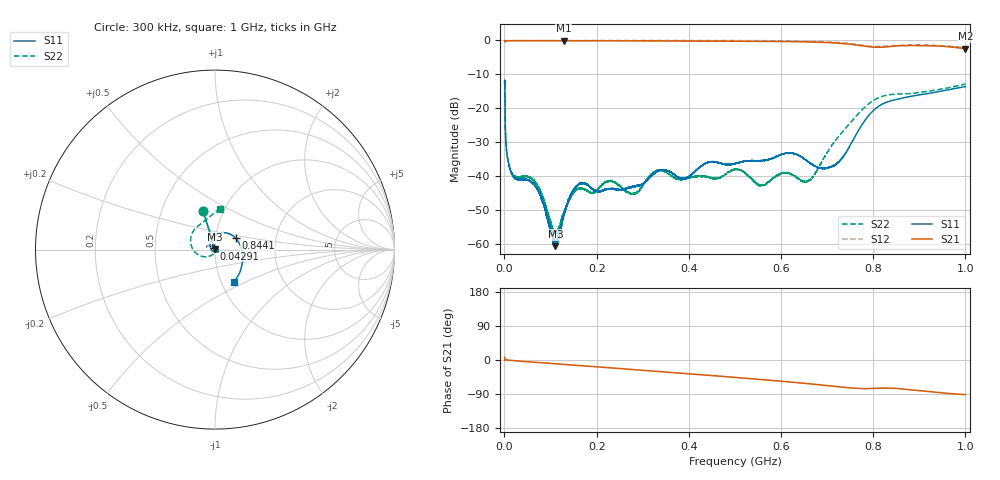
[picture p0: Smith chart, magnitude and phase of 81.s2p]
!Keysight Technologies,N5232A,MY52221221,A.10.65.11
!Date: Thursday, June 15, 2023 18:07:57
!Correction: S11(Full 2 Port(1,4))
!S41(Full 2 Port(1,4))
!S14(Full 2 Port(1,4))
!S44(Full 2 Port(1,4))
!S2P File: Measurements: S11, S41, S14, S44:
# Hz S  RI  R 50
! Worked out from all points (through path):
!   16001 points, 300 kHz to 1 GHz, reference 50 ohm
!   highest |S21| = -0.10 dB at 128.2 MHz (marker M1); lowest = -2.5 dB at 999.9 MHz (marker M2)
!   group delay of S21, straight-line fit = 257 ps
!   lowest |S11| = -60.7 dB at 110.5 MHz (marker M3), VSWR 1.00, Z = 50 + j0.0882 ohm
!   |S11| at or under -10 dB: start of sweep to end of sweep
!   |S22| runs from -57.1 to -11.7 dB; largest |S21 - S12| = 1.9
!   S11 on the Smith chart (normalised r, x): 300 kHz: 0.80, +0.36; 42.91 MHz: 0.99, +0.01; 844.1 MHz: 1.25, +0.16; 1 GHz: 1.14, -0.43
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300000  -0.0677 0.2157  0.9689 0.123  0.9368 0.1641  -0.0666 0.2135
6485644  -0.00905 0.0163  0.983 -0.00152  0.9859 0.0261  -0.00923 0.0157
1.135918e7  -0.00673 0.0111  0.9845 -0.0119  0.9867 0.0363  -0.00708 0.0111
4.291221e7  -0.00577 0.00669  0.9847 -0.0649  0.9829 0.1134  -0.0061 0.00771
7.390291e7  -0.00199 0.00555  0.9801 -0.1134  0.9699 0.1955  -0.00222 0.00647
1.105169e8  0.000265 0.000881  0.9699 -0.1712  0.9451 0.2868  -0.000701 0.00128
1.281991e8  0.000445 0.0025  0.9685 -0.1968  0.9349 0.3284  -0.000409 0.00272
1.669375e8  0.00407 0.00663  0.9493 -0.2557  0.8943 0.4244  0.00307 0.00574
2.304184e8  0.000491 0.00642  0.9182 -0.348  0.812 0.5682  -0.000926 0.00848
2.80216e8  0.00671 0.00157  0.8878 -0.4203  0.7328 0.6676  0.00404 0.00376
3.33575e8  0.0098 0.00684  0.8458 -0.4938  0.6333 0.7616  0.00777 0.00932
3.88621e8  0.00823 0.00364  0.7968 -0.5637  0.5174 0.8434  0.0041 0.00791
5.0015e8  0.0152 0.00135  0.6752 -0.697  0.2625 0.9539  0.00985 0.00775
5.541338e8  0.0154 -0.00667  0.6043 -0.7529  0.1364 0.9769  0.00658 0.00321
6.208013e8  0.0178 -0.013  0.5037 -0.8121  -0.0179 0.9742  0.00898 -0.00584
6.667875e8  0.007 -0.0131  0.4225 -0.8442  -0.1196 0.9538  0.00301 -0.00884
7.208963e8  -0.0115 -0.00994  0.3094 -0.8568  -0.2168 0.9058  -0.0178 -0.0304
7.904379e8  -0.00058 0.0785  0.2002 -0.7787  -0.3418 0.748  -0.1156 -0.00964
8.33425e8  0.0965 0.0792  0.2206 -0.7739  -0.4866 0.6713  -0.1258 0.0936
8.441093e8  0.1145 0.0641  0.2165 -0.7874  -0.5146 0.6605  -0.1145 0.1117
9.999375e8  0.1036 -0.1796  -0.0158 -0.7539  -0.6689 0.3963  0.0263 0.2244
1e9  0.1035 -0.1797  -0.0158 -0.7539  -0.6686 0.3965  0.0265 0.2244
